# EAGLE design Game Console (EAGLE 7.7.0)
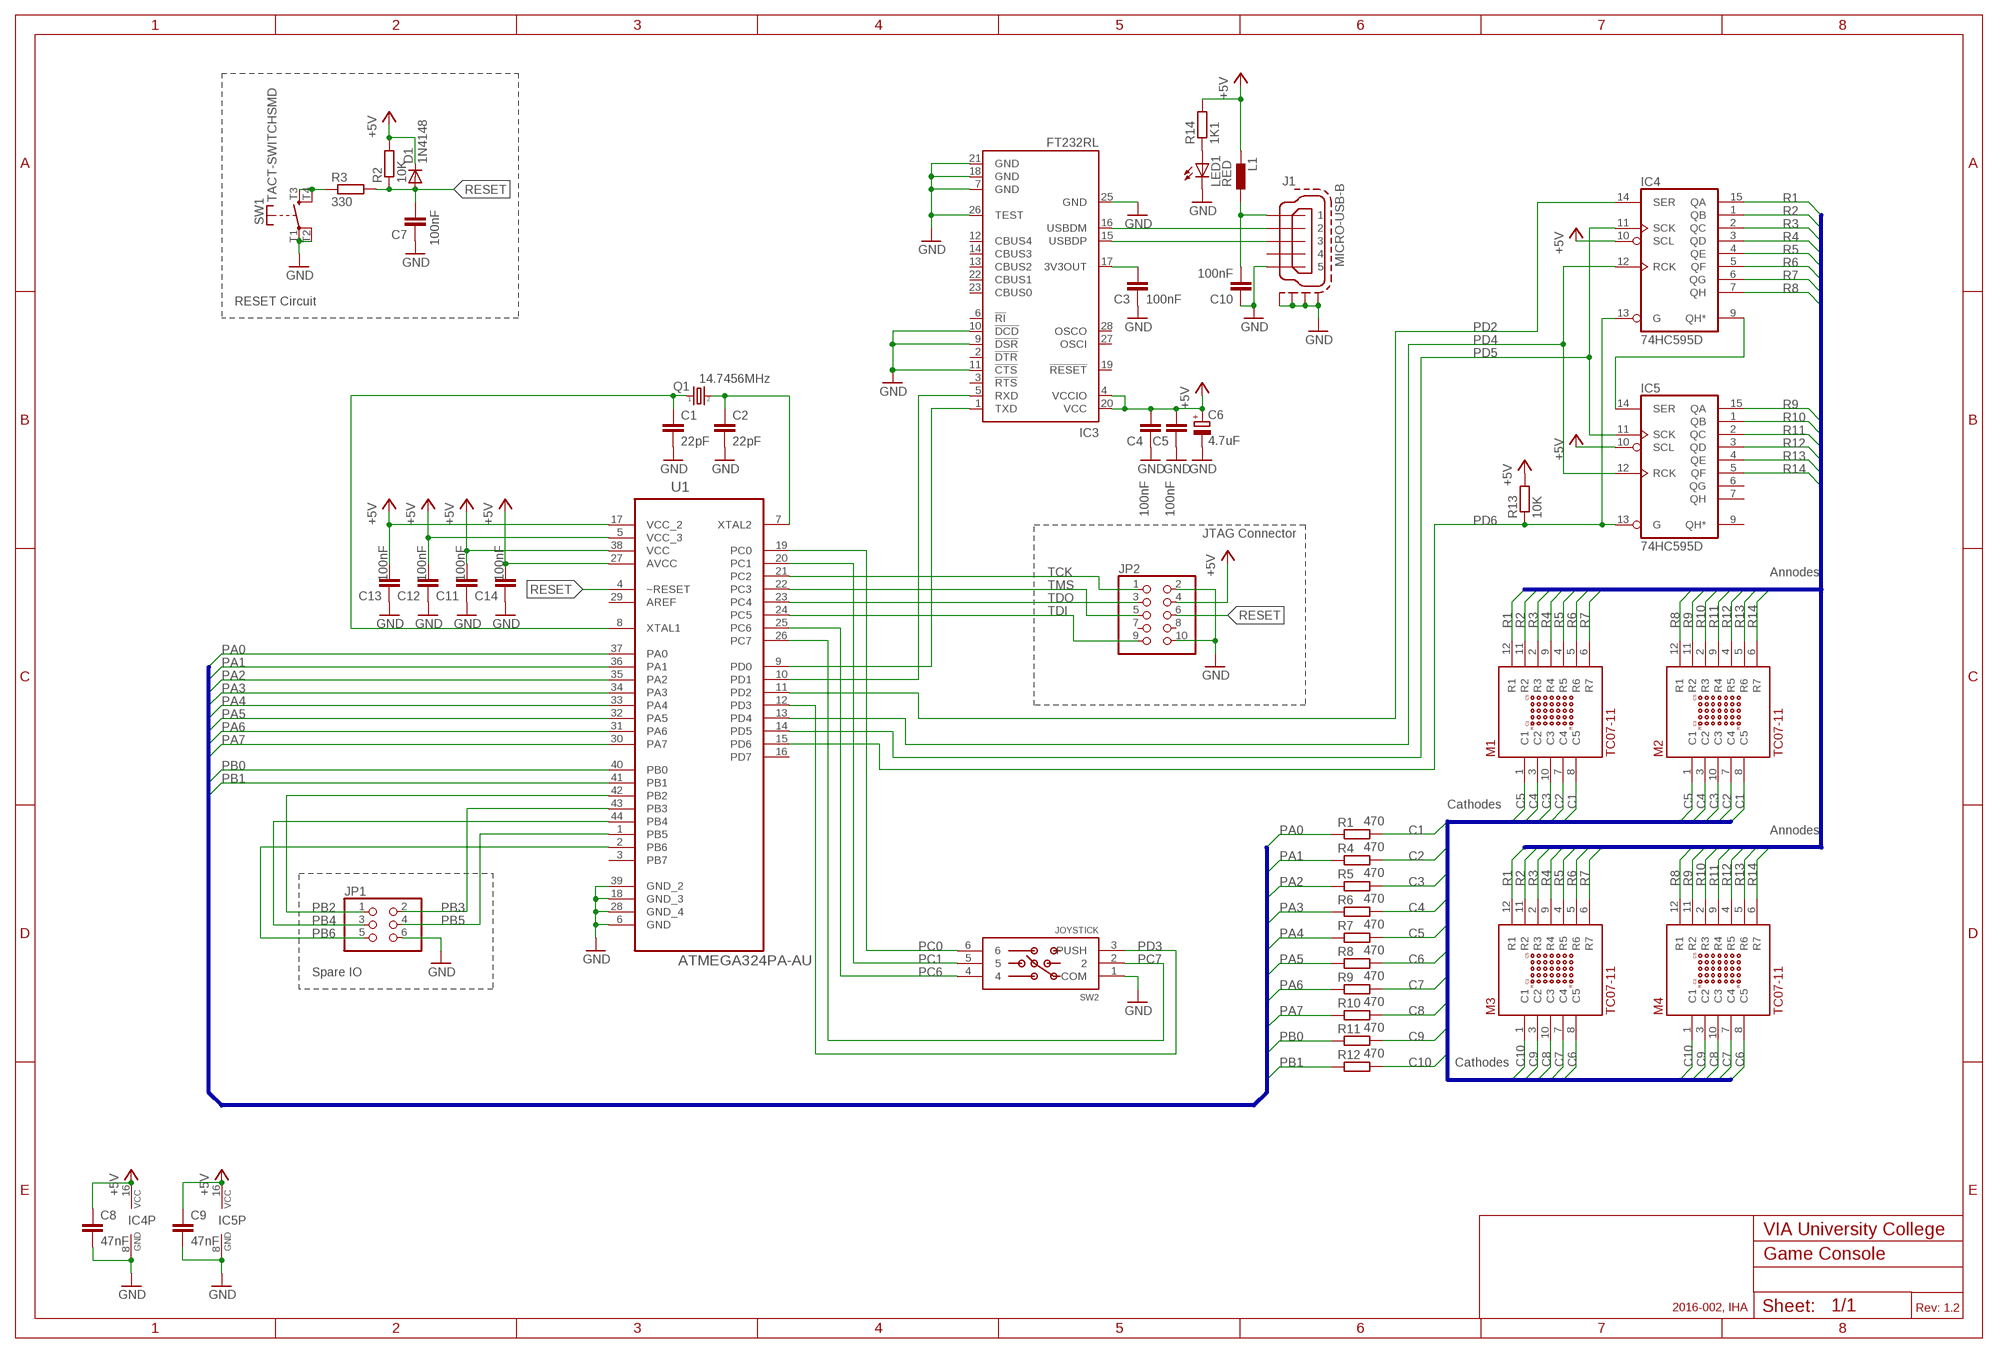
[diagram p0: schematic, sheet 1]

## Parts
C1  22pF  C-EUC0603  [C0603]
C2  22pF  C-EUC0603  [C0603]
C3  100nF  C-EUC0603  [C0603]
C4  100nF  C-EUC0603  [C0603]
C5  100nF  C-EUC0603  [C0603]
C6  4.7uF  CPOL-EUA/3216-18W  [A/3216-18W]
C7  100nF  C-EUC0603  [C0603]
C8  47nF  C-EUC0603  [C0603]
C9  47nF  C-EUC0603  [C0603]
C10  100nF  C-EUC0603  [C0603]
C11  100nF  C-EUC0603  [C0603]
C12  100nF  C-EUC0603  [C0603]
C13  100nF  C-EUC0603  [C0603]
C14  100nF  C-EUC0603  [C0603]
D1  1N4148  1N4148D0805  [D0805]
IC3  FT232RL  [SSOP28]
IC4  74HC595D  [SO16]
IC5  74HC595D  [SO16]
J1  MICRO-USB-B  [MOLEX-105017-0001]
JP1  PINHD-2X3  [2X03]
JP2  PINHD-2X5  [2X05]
L1  FERRITBEAD  [C0805]
LED1  RED  LEDCHIP-LED0805  [CHIP-LED0805]
M1  TC07-11  [TC07-11]
M2  TC07-11  [TC07-11]
M3  TC07-11  [TC07-11]
M4  TC07-11  [TC07-11]
Q1  14.7456MHz  X-TAL-C5CB  [C5CB]
R1  470  R-EU_R1206  [R1206]
R2  10K  R-EU_R1206  [R1206]
R3  330  R-EU_R1206  [R1206]
R4  470  R-EU_R1206  [R1206]
R5  470  R-EU_R1206  [R1206]
R6  470  R-EU_R1206  [R1206]
R7  470  R-EU_R1206  [R1206]
R8  470  R-EU_R1206  [R1206]
R9  470  R-EU_R1206  [R1206]
R10  470  R-EU_R1206  [R1206]
R11  470  R-EU_R1206  [R1206]
R12  470  R-EU_R1206  [R1206]
R13  10K  R-EU_R1206  [R1206]
R14  1K1  R-EU_R1206  [R1206]
SW1  TACT-SWITCHSMD  [DTSM-6]
SW2  JOYSTICK  [JS5208]
U1  ATMEGA324PA-AU  [QFP80P1200X1200X120-44N]

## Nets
+5V: C4.2 C5.2 C6.+ C8.1 C9.1 C11.2 C12.2 C13.2 C14.2 D1.C IC3.4(VCCIO) IC3.20(VCC) IC4.10(SCL) IC4.16(VCC) IC5.10(SCL) IC5.16(VCC) JP2.4 L1.1 R2.2 R13.2 R14.2 U1.5(VCC_3) U1.17(VCC_2) U1.27(AVCC) U1.38(VCC)
C1: M1.8(C5) M2.8(C5) R1.2
C2: M1.7(C4) M2.7(C4) R4.2
C3: M1.10(C3) M2.10(C3) R5.2
C4: M1.3(C2) M2.3(C2) R6.2
C5: M1.1(C1) M2.1(C1) R7.2
C6: M3.8(C5) M4.8(C5) R8.2
C7: M3.7(C4) M4.7(C4) R9.2
C8: M3.10(C3) M4.10(C3) R10.2
C9: M3.3(C2) M4.3(C2) R11.2
C10: M3.1(C1) M4.1(C1) R12.2
GND: C1.2 C2.2 C3.1 C4.1 C5.1 C6.- C7.1 C8.2 C9.2 C10.1 C11.1 C12.1 C13.1 C14.1 IC3.7(GND) IC3.9(!DSR) IC3.10(!DCD) IC3.11(!CTS) IC3.18(GND) IC3.21(GND) IC3.25(GND) IC3.26(TEST) IC4.8(GND) IC5.8(GND) J1.P$5 J1.P$6(S1) J1.P$7(S2) J1.P$8(S3) J1.P$9(S4) JP1.6 JP2.2 JP2.10 LED1.C SW1.T1(P) SW1.T2(P) SW2.1(COM) U1.6(GND) U1.18(GND_3) U1.28(GND_4) U1.39(GND_2)
N$1: C1.1 Q1.P$1 U1.8(XTAL1)
N$2: C2.1 Q1.P$2 U1.7(XTAL2)
N$3: IC4.9(QH*) IC5.14(SER)
N$4: IC3.1(TXD) U1.9(PD0)
N$5: IC3.5(RXD) U1.10(PD1)
N$6: C10.2 J1.P$1 L1.2
N$7: C3.2 IC3.17(3V3OUT)
N$11: IC3.16(USBDM) J1.P$2
N$12: IC3.15(USBDP) J1.P$3
N$14: R3.1 SW1.T3(S) SW1.T4(S)
N$17: LED1.A R14.1
PA0: R1.1 U1.37(PA0)
PA1: R4.1 U1.36(PA1)
PA2: R5.1 U1.35(PA2)
PA3: R6.1 U1.34(PA3)
PA4: R7.1 U1.33(PA4)
PA5: R8.1 U1.32(PA5)
PA6: R9.1 U1.31(PA6)
PA7: R10.1 U1.30(PA7)
PB0: R11.1 U1.40(PB0)
PB1: R12.1 U1.41(PB1)
PB2: JP1.1 U1.42(PB2)
PB3: JP1.2 U1.43(PB3)
PB4: JP1.3 U1.44(PB4)
PB5: JP1.4 U1.1(PB5)
PB6: JP1.5 U1.2(PB6)
PC0: SW2.6 U1.19(PC0)
PC1: SW2.5 U1.20(PC1)
PC6: SW2.4 U1.25(PC6)
PC7: SW2.2 U1.26(PC7)
PD2: IC4.14(SER) U1.11(PD2)
PD3: SW2.3(PUSH) U1.12(PD3)
PD4: IC4.12(RCK) IC5.12(RCK) U1.13(PD4)
PD5: IC4.11(SCK) IC5.11(SCK) U1.14(PD5)
PD6: IC4.13(G) IC5.13(G) R13.1 U1.15(PD6)
R1: IC4.15(QA) M1.12(R1) M3.12(R1)
R2: IC4.1(QB) M1.11(R2) M3.11(R2)
R3: IC4.2(QC) M1.2(R3) M3.2(R3)
R4: IC4.3(QD) M1.9(R4) M3.9(R4)
R5: IC4.4(QE) M1.4(R5) M3.4(R5)
R6: IC4.5(QF) M1.5(R6) M3.5(R6)
R7: IC4.6(QG) M1.6(R7) M3.6(R7)
R8: IC4.7(QH) M2.12(R1) M4.12(R1)
R9: IC5.15(QA) M2.11(R2) M4.11(R2)
R10: IC5.1(QB) M2.2(R3) M4.2(R3)
R11: IC5.2(QC) M2.9(R4) M4.9(R4)
R12: IC5.3(QD) M2.4(R5) M4.4(R5)
R13: IC5.4(QE) M2.5(R6) M4.5(R6)
R14: IC5.5(QF) M2.6(R7) M4.6(R7)
RESET: C7.2 D1.A JP2.6 R2.1 R3.2 U1.4(~RESET)
TCK: JP2.1 U1.21(PC2)
TDI: JP2.9 U1.24(PC5)
TDO: JP2.3 U1.23(PC4)
TMS: JP2.5 U1.22(PC3)
Unconnected: IC3.2(!DTR) IC3.3(!RTS) IC3.6(!RI) IC3.12(CBUS4) IC3.13(CBUS2) IC3.14(CBUS3) IC3.19(!RESET) IC3.22(CBUS1) IC3.23(CBUS0) IC3.27(OSCI) IC3.28(OSCO) IC5.6(QG) IC5.7(QH) IC5.9(QH*) J1.P$4 JP2.7 JP2.8 U1.3(PB7) U1.16(PD7) U1.29(AREF)

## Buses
C1,C2,C3,C4,C5,C6,C7,C8,C9,C10
R1,R2,R3,R4,R5,R6,R7,R8,R9,R10,R11,R12,R13,R14
PA0,PA1,PA2,PA3,PA4,PA5,PA6,PA7,PB0,PB1

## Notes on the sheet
- RESET Circuit
- JTAG Connector
- Annodes
- Cathodes
- Annodes
- Spare IO
- Cathodes
- VIA University College
- 2016-002, IHA
- Rev: 1.2

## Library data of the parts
C1-C5 C7-C14 = rcl:C-EU: CAPACITOR, European symbol
C6 = rcl:CPOL-EU: POLARIZED CAPACITOR, European symbol
D1 = IHA:1N4148: DIODE
IC3 = ftdichip:FT232R: Source: http://www.ftdichip.com/Documents/DataSheets/DS_FT232R_v104.pdf; MPN: FT232RL; OC_FARNELL: 1146032; OC_NEWARK: 91K9918
IC4 IC5 = 74xx-eu:74*595: 8-bit SHIFT REGISTER, output latch
J1 = IHA:MICRO-USB-B: Micro USB B Connector iha@via.dk; FARNELL: 2293836; MOLEX: 105017-0001
JP1 = pinhead:PINHD-2X3: PIN HEADER
JP2 = pinhead:PINHD-2X5: PIN HEADER
L1 = IHA:FERRITBEAD: Würths Electronics Chip Ferrite Bead
LED1 = led:LED: LED
M1-M4 = IHA:TC07-11: 5 x 7 LED Matrix LiteON: LTP-757KR iha@via.dk; DIGIKEY: 160-1555-5-ND
Q1 = IHA:X-TAL-C5CB: X-Tal QC5CB Series
R1-R14 = rcl:R-EU_: RESISTOR, European symbol
SW1 = IHA:TACT-SWITCH: Tact switch 6x6 mm Drawn by: Ib Havn iha@viauc.dk
SW2 = IHA:JOYSTICK: Joystick JS5208 E-Switch: JS5208 iha@via.dk; DIGIKEY: EG4561-ND
U1 = ATMEGA324:ATMEGA324PA-AU: 8-bit Microcontroller; MPN: ATMEGA324PA-AU; OC_FARNELL: 1715482; OC_NEWARK: 15R0265; PACKAGE: QFP-44; SUPPLIER: Atmel

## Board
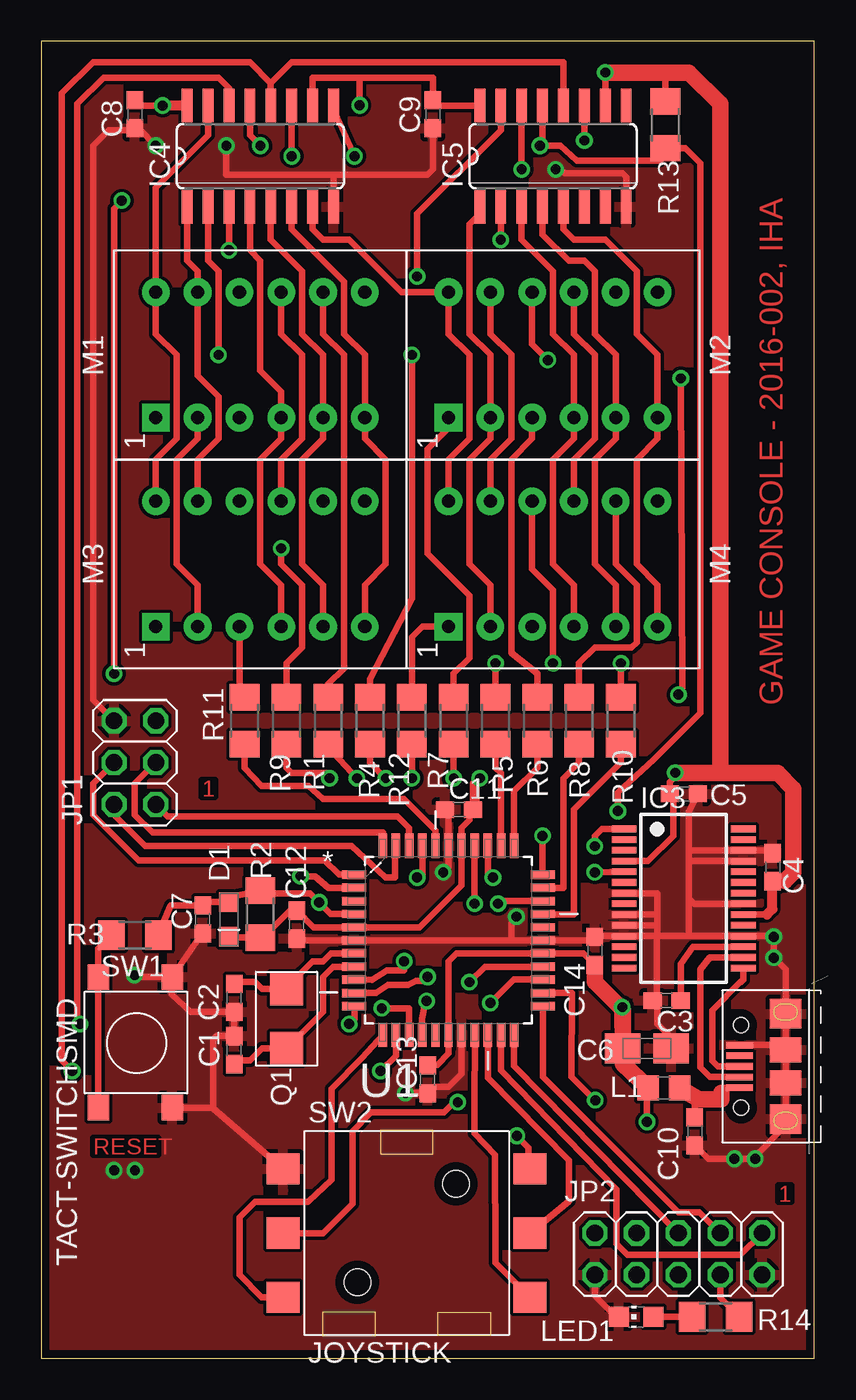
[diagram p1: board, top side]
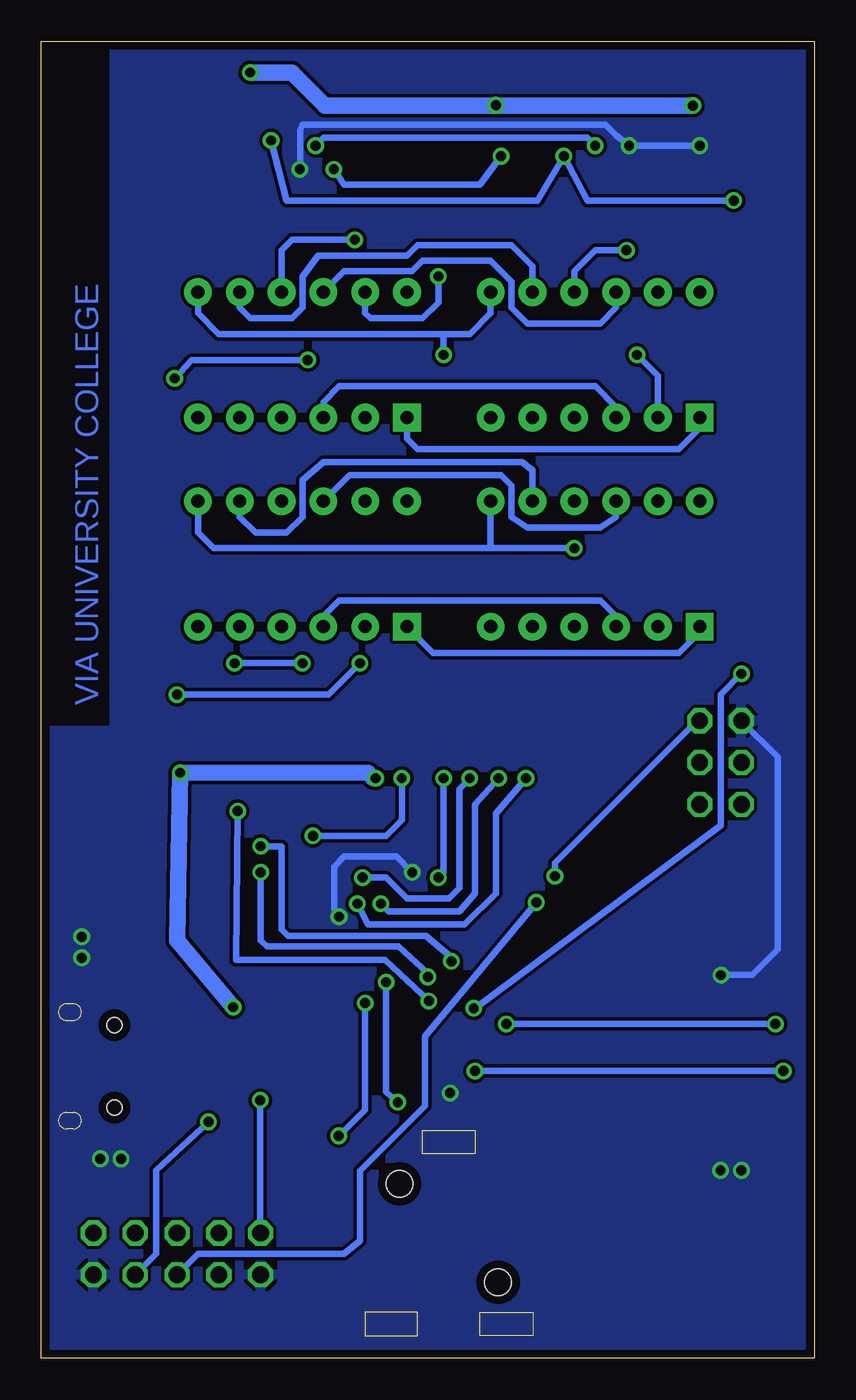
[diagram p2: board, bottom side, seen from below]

Size 46.97 x 80 mm. Coordinates in mm from the lower left corner, seen from the top.
Outline: 46.97,80 0,80 0,0 46.97,0 46.97,80
Copper layers (1*16): Top 0.035mm / dielectric 1.5mm / Bottom 0.035mm
Design rules "default *": minimum track width 10mil, minimum drill 23mil, track to track 8mil, track to pad 8mil, pad to pad 8mil, via to via 8mil, smd to smd 8mil, copper to edge 20mil, drill to drill 8mil, minimum pad ring 10mil, minimum via ring 8mil, stop-mask expansion 4mil, vias tented up to drill 0mil, thermal gap 10mil

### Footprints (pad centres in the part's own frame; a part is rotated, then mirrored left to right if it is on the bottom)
C0603 = smd 1.1 x 1: 1 -0.85,0; 2 0.85,0
A/3216-18W = smd 2.15 x 1.8: + 1.475,0; - -1.475,0
D0805 = smd 1.2 x 1.2: A 1.05,0; C -1.05,0
SSOP28 = smd 0.4 x 1.5: 1 -4.225,-3.625; 2 -3.575,-3.625; 3 -2.925,-3.625; 4 -2.275,-3.625; 5 -1.625,-3.625; 6 -0.975,-3.625; 7 -0.325,-3.625; 8 0.325,-3.625; 9 0.975,-3.625; 10 1.625,-3.625; 11 2.275,-3.625; 12 2.925,-3.625; 13 3.575,-3.625; 14 4.225,-3.625; 15 4.225,3.625; 16 3.575,3.625; 17 2.925,3.625; 18 2.275,3.625; 19 1.625,3.625; 20 0.975,3.625; 21 0.325,3.625; 22 -0.325,3.625; 23 -0.975,3.625; 24 -1.625,3.625; 25 -2.275,3.625; 26 -2.925,3.625; 27 -3.575,3.625; 28 -4.225,3.625
SO16 = smd 0.66 x 2.032: 1 -4.445,-3.073; 2 -3.175,-3.073; 3 -1.905,-3.073; 4 -0.635,-3.073; 5 0.635,-3.073; 6 1.905,-3.073; 7 3.175,-3.073; 8 4.445,-3.073; 9 4.445,3.073; 10 3.175,3.073; 11 1.905,3.073; 12 0.635,3.073; 13 -0.635,3.073; 14 -1.905,3.073; 15 -3.175,3.073; 16 -4.445,3.073
MOLEX-105017-0001 = smd 0.4 x 1.6: P$1 -1.3,2.8; P$2 -0.65,2.8; P$3 0,2.8; P$4 0.65,2.8; P$5 1.3,2.8 | smd 1.8 x 1.9: P$6 -3.2,0; P$9 3.2,0 | smd 1.5 x 1.9: P$7 -1,0; P$8 1,0 | hole 0.9: -2.5,2.7; 2.5,2.7
2X03 = drill 1.016 octagon: 1 -2.54,-1.27; 2 -2.54,1.27; 3 0,-1.27; 4 0,1.27; 5 2.54,-1.27; 6 2.54,1.27
2X05 = drill 1.016 octagon: 1 -5.08,-1.27; 2 -5.08,1.27; 3 -2.54,-1.27; 4 -2.54,1.27; 5 0,-1.27; 6 0,1.27; 7 2.54,-1.27; 8 2.54,1.27; 9 5.08,-1.27; 10 5.08,1.27
C0805 = smd 1.3 x 1.5: 1 -0.95,0; 2 0.95,0
CHIP-LED0805 = smd 1.2 x 1.2: A 0,-1.05; C 0,1.05
TC07-11 = drill 0.8 pad 1.676 square: 1 -3.81,6.35 | drill 0.8 pad 1.676: 2 -3.81,3.81; 3 -3.81,1.27; 4 -3.81,-1.27; 5 -3.81,-3.81; 6 -3.81,-6.35; 7 3.81,-6.35; 8 3.81,-3.81; 9 3.81,-1.27; 10 3.81,1.27; 11 3.81,3.81; 12 3.81,6.35
C5CB = smd 2 x 2: P$1 -1.8,0; P$2 1.8,0
R1206 = smd 1.6 x 1.803: 1 -1.422,0; 2 1.422,0
DTSM-6 = smd 1.549 x 1.295: T1 0,4.496; T2 7.95,4.496; T3 0,0; T4 7.95,0
JS5208 = smd 2 x 1.9: 1 -7.5,3.9; 2 -7.5,0; 3 -7.5,-3.9; 4 7.5,3.9; 5 7.5,0; 6 7.5,-3.9 | hole 1.6: 3,3; -3,-3
QFP80P1200X1200X120-44N = smd 1.473 x 0.508: 1 -5.74,3.988; 2 -5.74,3.2; 3 -5.74,2.388; 4 -5.74,1.6; 5 -5.74,0.787; 6 -5.74,0; 7 -5.74,-0.787; 8 -5.74,-1.6; 9 -5.74,-2.388; 10 -5.74,-3.2; 11 -5.74,-3.988; 23 5.74,-3.988; 24 5.74,-3.2; 25 5.74,-2.388; 26 5.74,-1.6; 27 5.74,-0.787; 28 5.74,0; 29 5.74,0.787; 30 5.74,1.6; 31 5.74,2.388; 32 5.74,3.2; 33 5.74,3.988 | smd 0.508 x 1.473: 12 -3.988,-5.74; 13 -3.2,-5.74; 14 -2.388,-5.74; 15 -1.6,-5.74; 16 -0.787,-5.74; 17 0,-5.74; 18 0.787,-5.74; 19 1.6,-5.74; 20 2.388,-5.74; 21 3.2,-5.74; 22 3.988,-5.74; 34 3.988,5.74; 35 3.2,5.74; 36 2.388,5.74; 37 1.6,5.74; 38 0.787,5.74; 39 0,5.74; 40 -0.787,5.74; 41 -1.6,5.74; 42 -2.388,5.74; 43 -3.2,5.74; 44 -3.988,5.74

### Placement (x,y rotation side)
C1  11.73,18.72 90 top
C2  11.73,21.89 270 top
C3  37.99,21.73 0 top
C4  44.43,29.83 270 top
C5  39.03,34.28 180 top
C6  36.8,18.83 180 top
C7  9.82,26.66 90 top
C8  5.7,75.55 270 top
C9  23.79,75.55 270 top
C10  39.71,13.78 90 top
C11  25.38,33.33 0 top
C12  15.54,26.34 90 top
C13  23.48,16.94 90 top
C14  33.63,24.75 270 top
D1  11.41,26.66 90 top
IC3  39.03,27.93 270 top
IC4  13.31,73.01 0 top
IC5  31.09,73.01 0 top
J1  45.22,17.73 90 top
JP1  5.7,36.18 90 top
JP2  38.71,6.34 180 top
L1  37.83,16.43 0 top
LED1  36.15,2.52 90 top
M1  13.31,60.95 90 top
M2  31.09,60.95 90 top
M3  13.31,48.25 90 top
M4  31.09,48.25 90 top
Q1  14.9,20.62 90 top
R1  17.44,38.72 90 top
R2  13.31,26.98 270 top
R3  5.7,25.71 0 top
R4  19.98,38.72 90 top
R5  27.6,38.72 90 top
R6  30.14,38.72 90 top
R7  25.06,38.72 90 top
R8  32.68,38.72 90 top
R9  14.9,38.72 90 top
R10  35.22,38.72 90 top
R11  12.36,38.72 90 top
R12  22.52,38.72 90 top
R13  37.92,74.92 90 top
R14  40.97,2.53 0 top
SW1  3.47,23.17 270 top
SW2  22.2,7.61 0 top
U1  24.74,25.39 0 top

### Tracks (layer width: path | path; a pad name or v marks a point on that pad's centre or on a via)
+5V  (via drill 0.6)
  Top 0.254: v38.52,35.57 38.66,35.52 38.71,35.55
  Top 0.406: C14.2 32.94,24.6 U1.27 25.23,24.6 24.74,24.12 U1.17 24.74,18.51 24.07,17.83 23.52,17.83 C13.2 | D1.C 11.46,25.55 R2.2 13.31,25.71 13.63,25.71 15.12,27.19 C12.2 16.55,26.17 U1.5 22.99,26.17 25.53,28.71 U1.38 25.53,32.21 26.02,32.69 26.02,33.11 C11.2 26.33,33.43 | IC3.20 44.09,26.95 | v7.38,76.09 6.01,76.09 C8.1 | IC5.16 24.11,76.09 C9.1 23.79,77.78 23.64,77.77 19.35,77.77 | IC4.10 16.49,77.78 16.81,77.77 19.35,77.77 | v19.35,76.11 19.35,77.77 | v34.27,78.09 IC5.10 | IC3.4 36.86,30.2 38.4,31.74 38.4,34.06 C5.2 | 38.08,34.38 C5.2 | R13.2 37.92,77.79 37.61,78.09 | v38.52,35.57 38.52,35.35 38.18,35.01 C5.2 | JP2.4 41.25,3.67 R14.2 | v36.8,14.36 36.8,16.42 L1.1 | 35.37,18.67 35.37,18.78 C6.+
  Top 0.61: 44.09,26.95 44.43,27.29 C4.2 45.17,28.98 | IC4.16 v7.38,76.09 | v26.65,35.23 26.33,34.91 26.33,33.43
  Top 1.016: L1.1 35.35,17.88 35.37,18.67 | 45.17,28.98 45.7,29.51 45.7,34.59 44.75,35.55 41.25,35.55 | 41.25,35.55 38.71,35.55 | v34.27,78.09 37.61,78.09 39.35,78.09 41.25,76.19 41.25,35.55 | v35.3,21.33 35.3,21.3 C6.+ 35.33,21.16 33.63,22.85 C14.2
  Bottom 0.254: v26.65,35.23 26.78,35.29 27.1,35.55
  Bottom 0.406: 20.83,76.09 v19.35,76.11 | JP2.4 39.98,6.34 39.98,11.42 v36.8,14.36
  Bottom 1.016: v7.38,76.09 20.83,76.09 29.72,76.09 31.73,78.09 v34.27,78.09 | 26.8,35.25 27.1,35.55 v38.52,35.57 38.71,25.39 35.37,21.41 v35.3,21.33
C1
  Top 0.406: R1.2 17.44,40.94 18.39,41.9 18.39,60.95 17.12,62.22 M1.8
  Bottom 0.406: M1.8 17.12,66.34 18.39,67.61 24.11,67.61 24.74,66.98 30.14,66.98 31.09,65.71 31.09,63.81 31.73,63.17 34.27,63.17 34.91,63.81 M2.8
C2  (via drill 0.6)
  Top 0.406: R4.2 19.98,41.26 22.54,46.16 22.54,60.8 v22.52,60.95
  Bottom 0.406: M1.7 19.66,63.49 20.94,62.22 22.52,62.22 | 22.52,62.22 36.17,62.22 37.45,63.49 M2.7 | v22.52,60.95 22.52,62.22
C3  (via drill 0.6)
  Top 0.406: M2.10 29.83,61.58 v30.78,60.63 | v38.86,59.52 38.94,40.7 v38.71,40.31 | v27.6,42.22 R5.2
  Bottom 0.406: M1.10 12.05,63.81 13,62.85 17.44,62.85 18.39,63.81 18.39,65.39 19.66,66.66 23.79,66.66 24.43,66.03 28.55,66.03 M2.10 | v30.78,60.63 37.83,60.63 v38.86,59.52 | v38.71,40.31 29.51,40.31 v27.6,42.22
C4
  Top 0.406: M2.3 29.83,55.87 28.55,54.6 28.55,42.85 30.14,41.58 R6.2
  Bottom 0.406: M1.3 12.05,57.77 13.31,59.04 28.87,59.04 29.83,58.09 M2.3
C5
  Top 0.406: M2.1 24.74,56.5 23.48,55.23 23.48,48.88 26.02,46.34 26.02,42.53 25.06,41.58 R7.2
  Bottom 0.406: M1.1 6.96,56.5 8.23,55.23 24.11,55.23 24.74,55.87 M2.1
C6
  Top 0.406: M4.8 34.91,48.25 36.17,46.98 36.17,43.48 35.86,43.17 33.63,43.17 32.68,42.22 R8.2
  Bottom 0.406: M3.8 17.12,53.96 17.76,54.44 29.83,54.44 31.09,53.33 31.09,51.11 32.05,50.15 33.95,50.15 34.91,51.11 M4.8
C7  (via drill 0.6)
  Top 0.406: R9.2 14.9,42.22 15.85,43.17 15.85,46.98 14.59,48.25 v14.59,49.2
  Bottom 0.406: M3.7 19.66,49.2 | 19.66,49.2 36.49,49.2 37.45,50.15 M4.7 | v14.59,49.2 19.66,49.2
C8  (via drill 0.6)
  Top 0.406: M4.10 29.83,47.93 31.09,46.66 v31.09,42.22 | v35.22,42.22 R10.2
  Bottom 0.406: M3.10 12.05,51.11 13,50.47 17.44,50.47 18.39,51.11 18.39,53.01 19.03,53.65 28.24,53.65 M4.10 | v31.09,42.22 v35.22,42.22
C9
  Top 0.406: M3.3 12.05,40.46 R11.2
  Bottom 0.406: M3.3 12.05,45.07 13,46.02 28.87,46.02 29.83,45.07 M4.3
C10
  Top 0.406: M4.1 23.16,44.44 22.52,43.8 R12.2
  Bottom 0.406: M3.1 6.96,44.12 8.23,42.85 23.16,42.85 M4.1
GND  (via drill 0.6)
  Top 0.406: C12.1 15.96,25.39 U1.6 28.55,25.39 | SW1.T1 9.72,25.71 C7.1 | IC3.9 37.42,26.95 | 37.42,26.95 37.45,26.98 37.45,28.24 35.41,28.24 IC3.7 | 37.39,25.65 IC3.11 33.69,25.65 C14.1 33.42,25.39 U1.28 28.55,25.39 | 37.39,25.65 37.45,25.71 37.45,26.34 | 37.45,26.34 37.45,26.93 37.42,26.95 | IC3.10 37.41,26.3 37.45,26.34 | C4.1 44.58,30.85 IC3.26 39.42,30.85 39.35,30.79 | 10.46,15.19 10.46,19.35 10.67,19.57 C1.2 C2.2 9.09,21.05 7.92,22.09 7.92,23.11 SW1.T1 | 10.46,15.19 SW2.1 | 39.35,25.65 IC3.18 44.45,25.65 v44.51,25.6 v44.51,24.33 45.22,23.62 J1.P$9 J1.P$8 | 39.35,25.65 37.39,25.65 | C11.1 24.74,33.11 U1.39 24.74,29.83 v24.43,29.51 | IC5.8 35.54,71.73 35.3,71.97 31.81,71.97 v31.25,72.22 | v11.25,73.65 11.25,71.9 17.76,71.9 | 17.76,71.9 IC4.8 | 17.76,71.9 23.48,71.9 23.79,72.22 C9.2 | 39.35,30.79 39.35,30.15 | 39.35,30.15 39.35,27.93 | 39.35,27.93 39.35,25.65 | IC3.21 39.67,27.6 39.35,27.93 | IC3.25 39.4,30.2 39.35,30.15 | v6.96,73.65 5.91,74.7 C8.2 5.59,74.6 4.11,74.6 3.16,73.65 3.16,39.99 JP1.6 | 39.35,30.79 39.35,33.22 C5.1 | 28.55,25.39 28.55,26.43 v28.87,26.82 | 37.39,25.65 37.39,22.05 C3.1 37.45,21.79 37.45,20.31 38.27,19.48 C6.- | SW1.T1 5.79,23.17 v5.68,23.27 | SW1.T2 10.43,15.21 10.46,15.19 | J1.P$5 44.92,19.03 J1.P$8 | J1.P$8 J1.P$7 J1.P$6 45.06,14.38 45.06,13.96 43.38,12.27 v43.38,12.12 v42.11,12.12 40.52,12.12 C10.1 | LED1.C 34.91,2.52 33.63,3.8 JP2.10 | U1.18 25.53,17.28 24.74,16.5 23.89,16.5 C13.1 | C13.1 23.07,16.09 | v22.12,16.11 23.46,16.11 C13.1
  Bottom 0.406: v6.96,73.65 v11.25,73.65 12.05,74.28 12.68,74.92 31.09,74.92 31.25,74.6 v31.25,72.22 | v28.87,26.82 28.87,26.98 29.19,27.29 29.19,29.83 28.55,30.47 25.38,30.47 v24.43,29.51 | v5.68,23.27 3.78,23.27 2.21,24.85 2.21,36.51 JP1.6
  other vias: 4.43,11.42 5.7,11.42
  pour Bottom: -0.66,80 42.53,80 42.53,38.09 47.61,38.09 47.61,-0.01 -0.66,-0.01
  pour Top: -0.66,80 42.53,80 42.53,38.09 47.61,38.09 47.61,-0.01 -0.66,-0.01
N$1
  Top 0.406: U1.8 17.75,23.79 17.12,23.17 17.12,21.05 Q1.P$1 13.42,18.83 12.68,18.08 11.94,18.08 C1.1
N$2
  Top 0.406: U1.7 17.61,24.6 17.12,24.12 16.49,24.12 15.85,23.48 Q1.P$2 13.42,22.42 13,22.85 11.83,22.85 C2.1
N$3  (via drill 0.6)
  Top 0.406: IC4.9 17.76,75.87 v19.03,73.01 | v29.19,72.22 IC5.14
  Bottom 0.406: v19.03,73.01 20.3,71.27 28.55,71.27 v29.19,72.22
N$4  (via drill 0.6)
  Top 0.406: U1.9 20.11,22.99 21.01,23.56 22.05,23.56 v22.05,24.12 | IC3.1 34.05,32.15 33.63,31.74 v33.63,31.1
  Bottom 0.406: v22.05,24.12 22.05,24.36 23.58,25.65 31.97,25.65 32.37,26.05 32.37,31.1 v33.63,31.1
N$5  (via drill 0.6)
  Top 0.406: U1.10 20.36,22.19 21.08,22.67 22.29,22.67 22.78,22.91 23.18,22.91 v23.48,23.17 | IC3.5 34.62,29.55 v33.63,29.51
  Bottom 0.406: v23.48,23.17 23.48,23.37 25.27,25.01 33.26,25.01 33.63,25.39 v33.63,29.51
N$6
  Top 0.406: C10.2 39.71,15.98 L1.2 | 42.34,16.43 J1.P$1 41.32,16.43 41.32,16.14
  Top 1.016: L1.2 39.95,15.73 41.32,15.73 41.32,16.14
N$7
  Top 0.406: IC3.17 39.6,25 38.87,23.95 38.87,21.76 C3.2
N$11
  Top 0.406: IC3.16 40.61,24.35 40.03,23.61 40.03,17.67 40.62,17.08 J1.P$2
N$12
  Top 0.406: IC3.15 42.66,22.98 42.53,22.85 42.47,22.85 40.76,21.14 40.76,18.07 41.1,17.73 J1.P$3
N$14
  Top 0.406: SW1.T4 SW1.T3 3.47,24.9 R3.1
N$17
  Top 0.406: LED1.A 39.54,2.52 R14.1
PA0  (via drill 0.6)
  Top 0.406: R1.1 17.44,37.13 v19.19,35.23 | v26.33,27.61 26.33,31.12 U1.37
  Bottom 0.406: v19.19,35.23 20.62,33.64 20.62,28.24 21.57,27.13 25.86,27.13 v26.33,27.61
PA1  (via drill 0.6)
  Top 0.406: R4.1 19.98,36.18 v20.94,35.23 | U1.36 27.13,29.36 v27.45,29.2
  Bottom 0.406: v20.94,35.23 21.57,34.59 21.57,28.56 22.2,27.93 24.74,27.93 26.01,29.2 v27.45,29.2
PA2
  Top 0.406: R5.1 27.6,35.87 27.92,35.55 27.92,31.15 U1.35
PA3
  Top 0.406: R6.1 30.14,35.87 28.73,34.46 U1.34
PA4  (via drill 0.6)
  Top 0.406: R7.1 v25.06,35.23 | v30.46,31.74 30.46,29.4 U1.33
  Bottom 0.406: v25.06,35.23 25.06,32.69 26.02,31.74 v30.46,31.74
PA5
  Top 0.406: R8.1 32.68,36.18 31.73,35.23 31.73,28.56 30.51,28.56 U1.32
PA6  (via drill 0.6)
  Top 0.406: R9.1 14.9,35.87 15.22,35.55 17.44,35.55 v17.52,35.23 | U1.31 27.84,27.78 v27.76,27.61
  Bottom 0.406: v17.52,35.23 19.35,33.08 19.35,28.24 21.25,26.34 27.12,26.34 v27.76,27.61
PA7
  Top 0.406: R10.1 35.22,36.18 32.37,33.33 32.37,26.98 30.5,26.98 U1.30
PB0
  Top 0.406: R11.1 12.36,35.87 13.39,34.76 16.25,34.76 17.12,33.96 22.04,33.96 23.96,32.05 U1.40
PB1  (via drill 0.6)
  Top 0.406: R12.1 v22.52,35.23 | v22.84,29.2 23.16,29.2 23.16,31.12 U1.41
  Bottom 0.406: v22.52,35.23 22.52,29.51 v22.84,29.2
PB2
  Top 0.406: U1.42 22.36,32.2 21.65,32.91 7.7,32.91 JP1.1
PB3
  Top 0.406: U1.43 21.48,31.07 21.48,29.2 20.94,29.2 18.86,31.11 10.47,31.11 6.32,31.11 4.43,33.01 JP1.2
PB4
  Top 0.406: U1.44 20.76,31.94 6.76,31.94 5.7,33.01 5.7,34.91 JP1.3
PB5
  Top 0.406: U1.1 18.09,29.38 17.21,30.25 5.91,30.25 3.16,33.01 3.16,34.91 JP1.4
PB6  (via drill 0.6)
  Top 0.406: v15.76,29.28 16.65,29.28 17.45,28.56 18.97,28.56 U1.2
  Bottom 0.406: JP1.5 7.12,38.72 15.76,30.09 v15.76,29.28
PC0
  Top 0.406: U1.19 26.34,18.07 26.33,16.82 26.33,13.67 27.55,12.35 27.6,6.45 27.6,5.81 SW2.6
PC1
  Top 0.406: U1.20 27.13,17.02 32.05,12.02 32.05,9.55 SW2.5
PC6  (via drill 0.6)
  Top 0.406: U1.25 28.71,23 v27.28,21.58 | SW2.4 29.62,11.42 29.62,12.8 v28.9,13.51
  Bottom 0.406: v27.28,21.58 27.29,15.09 28.87,13.51 v28.9,13.51
PC7  (via drill 0.6)
  Top 0.406: U1.26 26.95,23.79 v26.02,22.85 | SW2.2 17.12,7.61 18.9,9.39 18.9,13.8 20.03,14.93 24.47,14.93 25.09,15.55 v25.31,15.55
  Bottom 0.406: v26.02,22.85 26.02,16.17 v25.31,15.55
PD2  (via drill 0.6)
  Top 0.406: IC4.14 11.41,77.14 10.77,77.78 3.79,77.78 2.2,76.19 2.2,20.31 v2.36,20.31 | v18.71,20.31 19.03,20.62 19.03,21.37 U1.11
  Bottom 0.406: v2.36,20.31 14.59,20.31 v18.71,20.31
PD3
  Top 0.406: SW2.3 13.41,3.71 12.05,5.07 12.05,8.56 13,9.51 16.17,9.51 16.24,9.52 17.63,10.83 17.63,16.38 19.51,18.24 20.78,19.65 U1.12
PD4  (via drill 0.6)
  Top 0.406: U1.13 21.55,18.36 v20.62,17.45 | v1.88,17.45 1.25,18.08 1.25,76.82 3.16,78.73 12.68,78.73 13.95,77.46 | IC5.12 31.73,78.73 15.22,78.73 13.95,77.46 | IC4.12 13.95,77.46
  Bottom 0.406: v20.62,17.45 v1.88,17.45
PD5  (via drill 0.6)
  Top 0.406: U1.14 22.36,21.27 v20.69,21.26 | v4.43,41.58 4.43,69.84 v4.9,70.31 | v15.22,73.01 IC4.11 | v33,73.97 IC5.11
  Bottom 0.406: v20.69,21.26 20.62,21.26 5.7,32.37 5.7,40.31 v4.43,41.58 | v4.9,70.31 13.79,70.31 v15.22,73.01 16.81,70.31 32.05,70.31 v33,73.97
PD6  (via drill 0.6)
  Top 0.406: IC5.13 30.46,73.81 v30.3,73.65 31.55,73.65 32.53,72.75 37.58,72.75 R13.1 39.13,73.5 40.03,72.59 40.03,39.2 37.21,36.38 | v13.31,73.65 12.68,74.28 IC4.13 | 37.21,36.38 | 37.21,36.38 35.03,34.36 v35.03,33.23 | v23.42,21.7 23.34,21.7 23.14,20.62 U1.15
  Bottom 0.406: v30.3,73.65 29.83,74.12 13.79,74.12 v13.31,73.65 | v23.42,21.7 26.08,24.2 35.11,24.2 v35.03,33.23
R1
  Top 0.406: M3.12 6.96,54.6 8.23,55.87 8.23,60.95 6.96,62.22 M1.12 6.96,71.11 10.14,74.28 IC4.15
R2
  Top 0.406: IC4.1 8.87,66.66 9.51,66.03 M1.11 9.51,59.68 10.77,58.41 10.77,55.87 9.51,54.6 M3.11
R3  (via drill 0.6)
  Top 0.406: IC4.2 10.14,66.66 10.77,66.03 v10.77,60.95 | M1.2 9.51,55.87 8.23,54.6 8.23,48.25 9.51,46.98 M3.2
  Bottom 0.406: v10.77,60.95 9.51,59.68 M1.2
R4  (via drill 0.6)
  Top 0.406: M1.9 14.59,62.22 15.85,60.95 15.85,55.87 14.59,54.6 M3.9 | IC4.3 v11.41,67.3
  Bottom 0.406: v11.41,67.3 13.31,67.3 14.59,66.03 M1.9
R5
  Top 0.406: IC4.4 12.68,67.3 13.31,66.66 13.31,60 14.59,58.73 M1.4 14.59,55.87 13.31,54.6 13.31,48.25 14.59,46.98 M3.4
R6
  Top 0.406: IC4.5 13.95,67.93 15.85,66.03 15.85,62.22 17.12,60.95 M1.5 17.12,55.87 15.85,54.6 15.85,48.25 17.12,46.98 M3.5
R7
  Top 0.406: IC4.6 15.22,68.57 18.39,65.39 18.39,62.22 19.66,60.95 M1.6 19.66,55.87 20.94,54.6 20.94,48.25 19.66,46.98 M3.6
R8
  Top 0.406: M4.12 24.74,54.6 26.02,55.87 26.02,60.95 24.74,62.22 M2.12 21.89,64.76 18.71,67.93 17.12,67.93 16.49,68.57 IC4.7
R9  (via drill 0.6)
  Top 0.406: M2.11 27.28,62.22 28.55,60.95 28.55,55.87 27.28,54.6 M4.11 | IC5.15 27.92,74.6 22.84,69.52 v22.84,65.71
  Bottom 0.406: v22.84,65.71 22.84,64.12 23.79,63.17 26.97,63.17 27.28,63.49 M2.11
R10
  Top 0.406: IC5.1 26.65,69.52 26.02,68.89 26.02,62.22 27.28,60.95 M2.2 27.28,55.87 26.02,54.6 26.02,48.25 27.28,46.98 M4.2
R11  (via drill 0.6)
  Top 0.406: IC5.2 v27.92,67.93 | M2.9 32.37,62.22 33.63,60.95 33.63,55.87 32.37,54.6 M4.9
  Bottom 0.406: v27.92,67.93 31.73,67.93 32.37,67.3 M2.9
R12
  Top 0.406: IC5.3 29.19,67.93 31.09,66.03 31.09,62.22 32.37,60.95 M2.4 32.37,55.87 31.09,54.6 31.09,48.25 32.37,46.98 M4.4
R13
  Top 0.406: IC5.4 30.46,68.25 32.05,66.66 33,66.66 33.63,66.03 33.63,62.22 34.91,60.95 M2.5 34.91,55.87 33.63,54.6 33.63,48.25 34.91,46.98 M4.5
R14
  Top 0.406: IC5.5 31.73,68.57 32.37,67.93 34.27,67.93 36.17,66.03 36.17,62.22 37.45,60.95 M2.6 37.45,55.87 36.17,54.6 36.17,48.25 37.45,46.98 M4.6
RESET  (via drill 0.6)
  Top 0.406: R3.2 7.85,27.51 C7.2 10.02,27.71 D1.A 11.78,28.08 R2.1 13.33,28.4 13.48,28.24 16.33,28.24 v16.89,27.69 17.59,26.99 U1.4
  Bottom 0.406: JP2.6 37.45,6.34 28.55,6.34 27.61,7.12 27.61,11.38 23.66,15.33 23.66,19.55 v16.89,27.69
TCK
  Top 0.406: JP2.1 42.49,6.3 35.6,6.3 34.95,6.94 34.95,10.25 27.95,17.5 U1.21
TDI  (via drill 0.6)
  Top 0.406: U1.24 32.23,22.19 32.21,17.1 33.64,15.67 v33.66,15.67
  Bottom 0.406: v33.66,15.67 33.66,7.63 JP2.9
TDO
  Top 0.406: U1.23 30.48,17.11 38.71,8.88 39.98,8.88 JP2.3
TMS
  Top 0.406: U1.22 28.73,17.75 JP2.5

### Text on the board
Top: GAME CONSOLE - 2016-002, IHA | 1 | RESET | 1
Bottom: VIA UNIVERSITY COLLEGE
